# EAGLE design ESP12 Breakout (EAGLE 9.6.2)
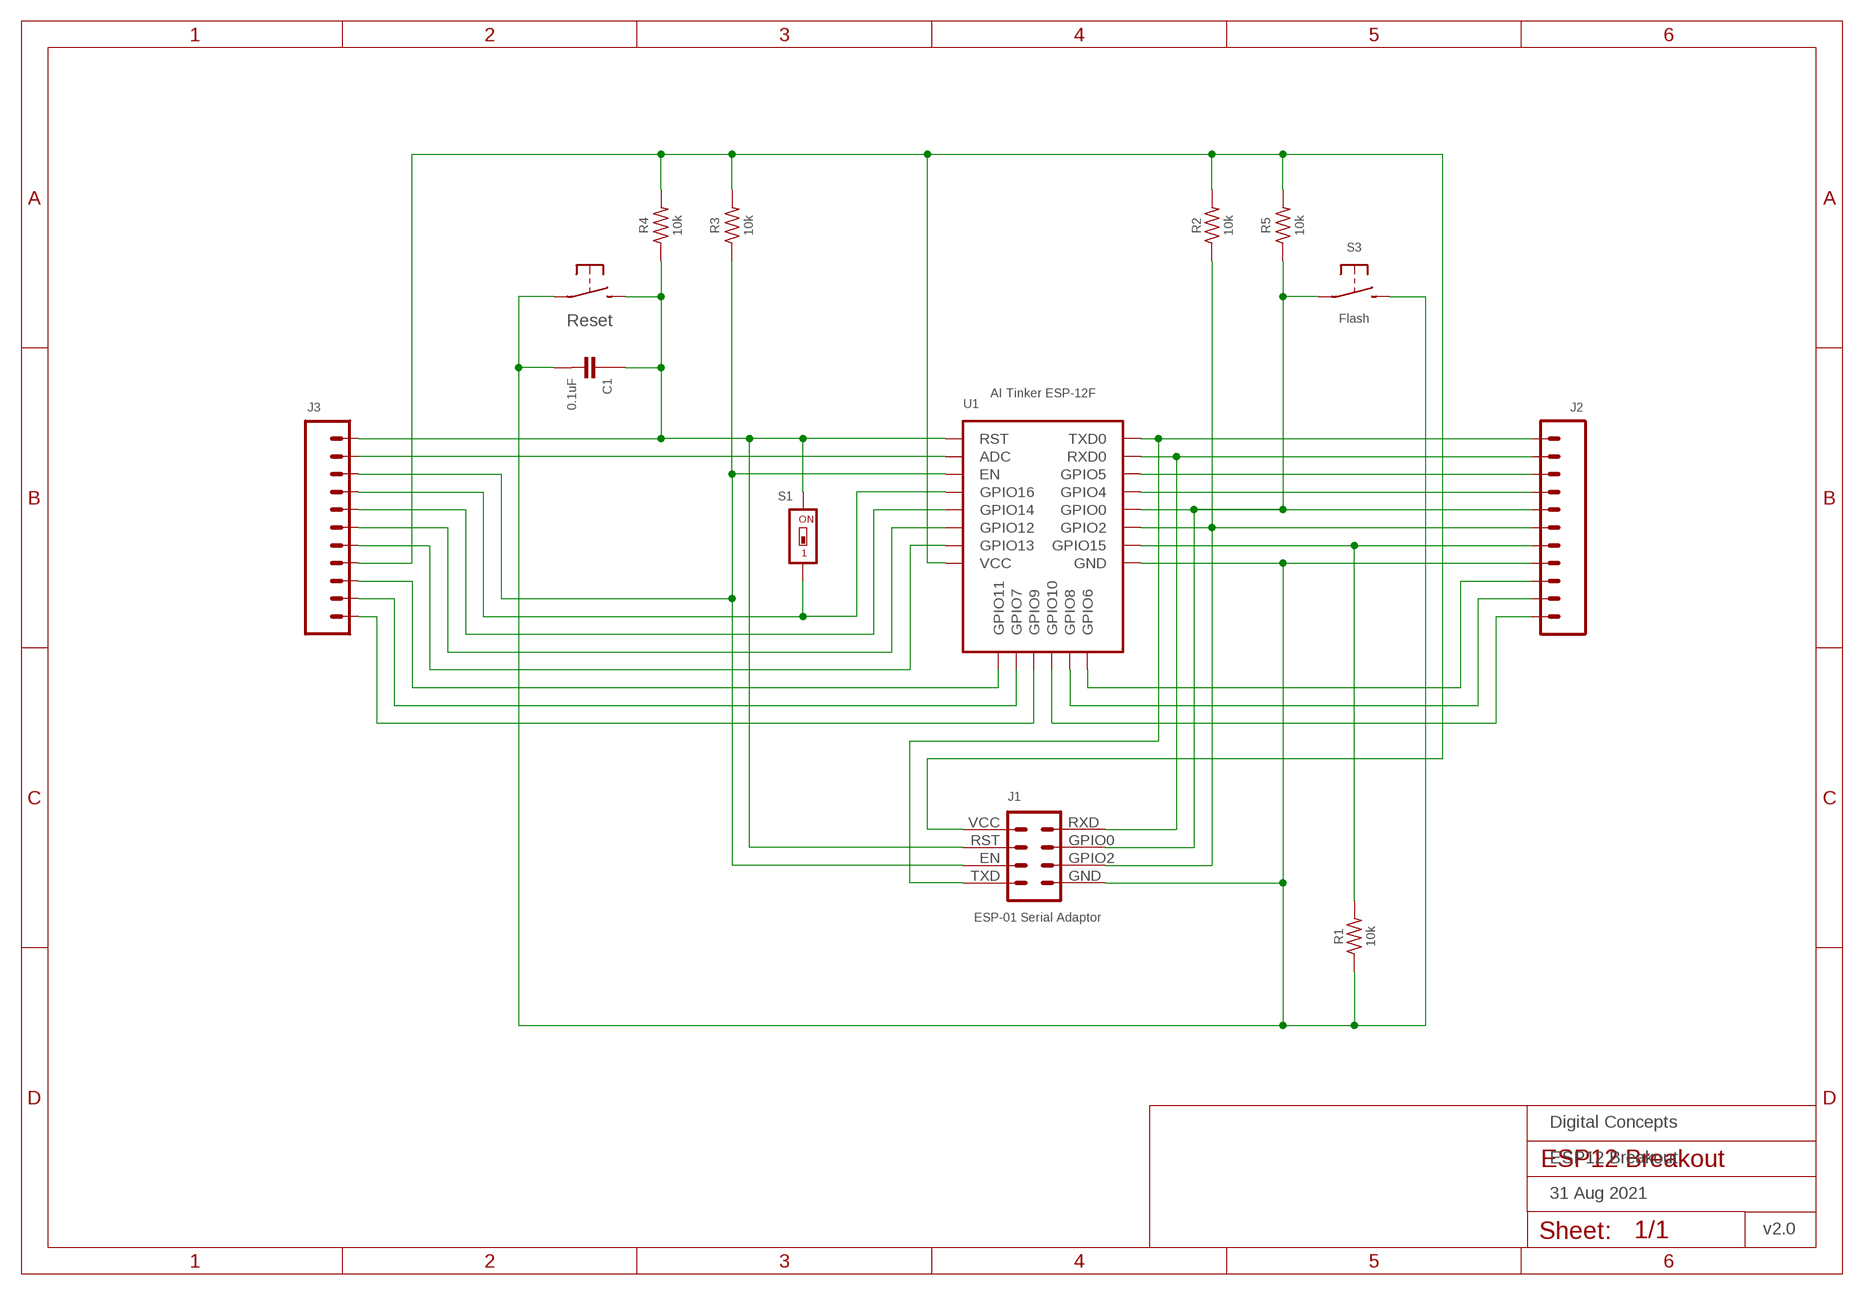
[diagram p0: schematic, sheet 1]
FRAME1 (A4L-LOC): DATE: 31 Aug 2021; OWNER: Digital Concepts; TITLE: ESP12 Breakout; VERSION: v2.0

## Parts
C1  0.1uF  CAPACITOR-0805  [C0805]
J1  ESP-01 Serial Adaptor  ESP-01-SERIAL-ADAPTOR  [CONN_2X4-ESP-01-SERIAL]
J2  HEADER-1X11-GENERIC  [CONN_11-GENERIC]
J3  HEADER-1X11-GENERIC  [CONN_11-GENERIC]
R1  10k  RESISTORR0805  [R0805]
R2  10k  RESISTORR0805  [R0805]
R3  10k  RESISTORR0805  [R0805]
R4  10k  RESISTORR0805  [R0805]
R5  10k  RESISTORR0805  [R0805]
S1  Wake  SWITCH-DIP-SWS001  [SMD-001]
S2  Reset  SWITCH-MOMENTARY-2-PIN  [SWITCH-2-PAD]
S3  Flash  SWITCH-MOMENTARY-2-PIN  [SWITCH-2-PAD]
U1  AI Tinker ESP-12F  ESP-12E/F  [ESP-12E/F]

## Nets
GND: C1.2 J1.GND J2.4 R1.1 S2.P$1(P) S3.P$2(S) U1.GND
N$1: J3.1 U1.GPIO9
N$2: J2.5 R1.2 U1.GPIO15
N$3: J3.7 U1.GPIO14
N$4: C1.1 J1.RST J3.11 R4.1 S1.2 S2.P$2(S) U1.RST
N$5: J3.6 U1.GPIO12
N$6: J3.5 U1.GPIO13
N$7: J3.10 U1.ADC
N$8: J1.EN J3.9 R3.1 U1.EN
N$9: J2.9 U1.GPIO5
N$10: J1.TXD J2.11 U1.TXD0
N$11: J1.GPIO2 J2.6 R2.1 U1.GPIO2
N$12: J2.8 U1.GPIO4
N$13: J1.GPIO0 J2.7 R5.1 S3.P$1(P) U1.GPIO0
N$15: J2.1 U1.GPIO10
N$16: J1.RXD J2.10 U1.RXD0
N$17: J2.3 U1.SCLK(GPIO6)
N$18: J3.8 S1.1 U1.GPIO16
N$19: J2.2 U1.MOSI(GPIO8)
N$22: J3.3 U1.CS0(GPIO11)
N$23: J3.2 U1.MISO(GPIO7)
VCC: J1.VCC J3.4 R2.2 R3.2 R4.2 R5.2 U1.VCC

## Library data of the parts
C1 = digitalconcepts:CAPACITOR-0805: 0805 Capacitor
J1 = digitalconcepts:ESP-01-SERIAL-ADAPTOR: ESP-01 Serial Adpator
J2 J3 = digitalconcepts:HEADER-1X11-GENERIC: Single Row 11-Pin Header
R1-R5 = digitalconcepts:RESISTOR: Resistor; SPICEPREFIX: R
S1 = digitalconcepts:SWITCH-DIP-SWS001: SMD Dip Switch 1 pol.
S2 S3 = digitalconcepts:SWITCH-MOMENTARY-2-PIN: 2 Pin Momentary Switch
U1 = digitalconcepts:ESP-12E/F: AI Thinker ESP-12E/F MCU

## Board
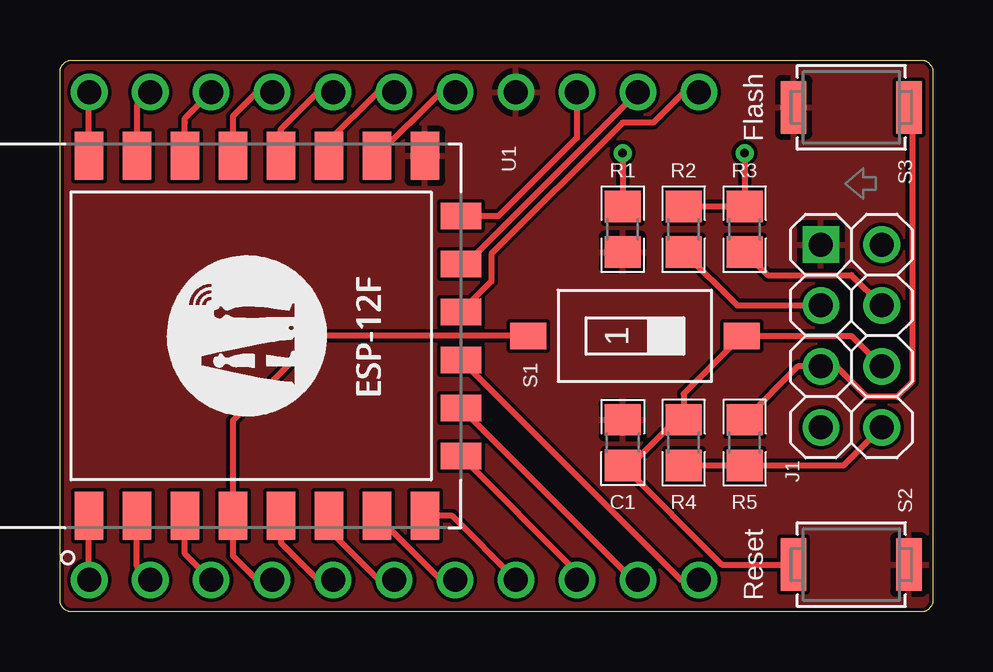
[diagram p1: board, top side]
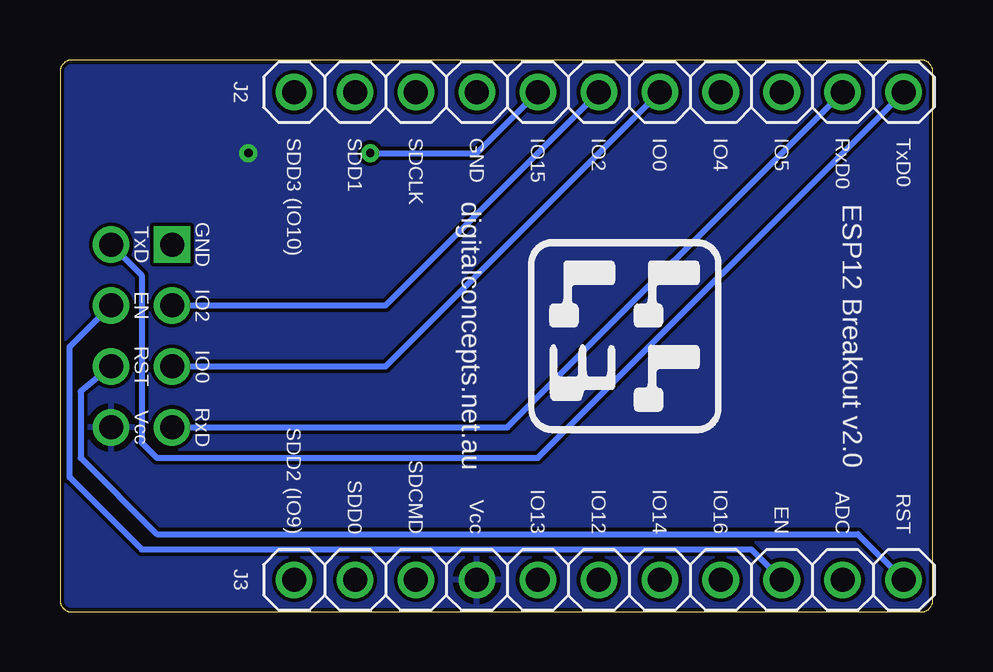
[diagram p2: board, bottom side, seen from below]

Size 36.37 x 23 mm. Coordinates in mm from the lower left corner, seen from the top.
Outline: 88 segments
Copper layers (1*16): Top 0.035mm / dielectric 1.5mm / Bottom 0.035mm
Design rules "default *": minimum track width 6mil, minimum drill 0.35mm, track to track 6mil, track to pad 6mil, pad to pad 6mil, via to via 6mil, smd to smd 6mil, copper to edge 6mil, drill to drill 6mil, minimum pad ring 10mil, minimum via ring 8mil, stop-mask expansion 4mil, vias tented up to drill 0mil, thermal gap 10mil

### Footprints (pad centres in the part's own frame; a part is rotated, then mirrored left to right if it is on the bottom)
C0805 = smd 1.3 x 1.5: 1 -0.95,0; 2 0.95,0
CONN_2X4-ESP-01-SERIAL = drill 1 pad 1.524: EN 2.54,2.54; GPIO0 5.08,0; GPIO2 2.54,0; RST 5.08,2.54; RXD 7.62,0; TXD 0,2.54; VCC 7.62,2.54 | drill 1 pad 1.524 square: GND 0,0
CONN_11-GENERIC = drill 1 pad 1.524: 1 0,0; 2 2.54,0; 3 5.08,0; 4 7.62,0; 5 10.16,0; 6 12.7,0; 7 15.24,0; 8 17.78,0; 9 20.32,0; 10 22.86,0; 11 25.4,0
R0805 = smd 1.3 x 1.5: 1 -0.95,0; 2 0.95,0
SMD-001 = smd 1.1 x 1.5: 1 0,-4.45; 2 0,4.45
SWITCH-2-PAD = smd 1.067 x 2.184: P$1 -2.4,0; P$2 2.4,0
ESP-12E/F = smd 2 x 1.2: ADC -7.5,5; EN -7.5,3; GND 7.5,-7; GPIO0 7.5,-1; GPIO2 7.5,-3; GPIO4 7.5,1; GPIO5 7.5,3; GPIO12 -7.5,-3; GPIO13 -7.5,-5; GPIO14 -7.5,-1; GPIO15 7.5,-5; GPIO16 -7.5,1; RST -7.5,7; RXD0 7.5,5; TXD0 7.5,7; VCC -7.5,-7 | smd 1.1 x 1.7: CS0 -5,-8.5; GPIO9 -1,-8.5; GPIO10 1,-8.5; MISO -3,-8.5; MOSI 3,-8.5; SCLK 5,-8.5

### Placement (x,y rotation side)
C1  23.44,7.06 90 top
J1  31.7,15.31 270 top
J2  26.62,21.66 0 bottom
J3  26.62,1.34 0 bottom
R1  23.44,15.95 90 top
R2  25.98,15.95 90 top
R3  28.52,15.95 90 top
R4  25.98,7.06 270 top
R5  28.52,7.06 270 top
S1  23.95,11.5 270 top
S2  32.97,1.98 180 top
S3  32.97,21.03 180 top
U1  8.2,11.5 90 top

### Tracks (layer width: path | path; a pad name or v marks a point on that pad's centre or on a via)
GND
  pour Top (rank 3): -1.32,24.2 37.41,24.2 37.41,-1.2 -1.32,-1.2
N$1
  Top 0.254: U1.GPIO9 25.86,1.34 J3.1
N$2  (via drill 0.35)
  Top 0.254: U1.GPIO15 15.86,21.66 J2.5 | v23.44,19.12 R1.2
  Bottom 0.254: J2.5 19,19.12 v23.44,19.12
N$3
  Top 0.254: U1.GPIO14 9.2,2.88 10.74,1.34 J3.7
N$4
  Top 0.254: J1.RST 32.97,11.5 S1.2 25.98,9.08 R4.1 25.68,8.01 23.78,6.11 C1.1 27.57,1.98 S2.P$2 | J3.11 1.2,1.36 U1.RST
  Bottom 0.254: J1.RST 35.51,9.19 35.51,6.42 32.33,3.25 3.12,3.25 J3.11
N$5
  Top 0.254: U1.GPIO12 11.2,3.42 13.28,1.34 J3.6
N$6
  Top 0.254: U1.GPIO13 15.86,1.34 J3.5
N$7
  Top 0.254: U1.ADC 3.2,1.9 J3.10
N$8
  Top 0.254: R3.1 29.48,14.04 32.97,14.04 J1.EN | U1.EN 5.2,2.44 J3.9
  Bottom 0.254: J1.EN 35.97,11.04 35.97,5.61 32.97,2.61 7.57,2.61 J3.9
N$9
  Top 0.254: U1.GPIO5 5.2,20.39 5.2,20.57 J2.9
N$10
  Top 0.254: U1.TXD0 1.2,21.65 J2.11
  Bottom 0.254: J1.TXD 32.97,14.04 32.97,7.06 32.33,6.42 16.46,6.42 J2.11
N$11
  Top 0.254: U1.GPIO2 11.2,19.64 13.23,21.66 J2.6 | R2.1 28.21,12.77 J1.GPIO2
  Bottom 0.254: J1.GPIO2 22.81,12.77 J2.6
N$12
  Top 0.254: U1.GPIO4 7.2,20.66 8.2,21.66 J2.8
N$13
  Top 0.254: U1.GPIO0 9.2,20.12 | 9.2,20.12 | 9.2,20.12 10.74,21.66 J2.7 | R5.1 30.75,10.23 J1.GPIO0 32.33,10.23 33.6,8.96 34.87,8.96 35.51,9.6 35.51,20.89 S3.P$1
  Bottom 0.254: J1.GPIO0 22.81,10.23 J2.7
N$15
  Top 0.254: U1.GPIO10 17.97,13.77 17.97,14.92 23.44,20.39 24.71,20.39 25.98,21.66 J2.1
N$16
  Top 0.254: U1.RXD0 3.2,21.11 J2.10
  Bottom 0.254: J1.RXD 17.73,7.69 J2.10
N$17
  Top 0.254: U1.SCLK 18.28,16.5 21.54,19.76 J2.3
N$18
  Top 0.254: S1.1 10.74,11.5 7.2,7.96 U1.GPIO16 7.2,2.34 8.2,1.34 J3.8
N$19
  Top 0.254: J2.2 16.92,14.5 U1.MOSI
N$22
  Top 0.254: U1.CS0 21.54,1.67 J3.3
N$23
  Top 0.254: U1.MISO 23.86,1.34 J3.2
VCC  (via drill 0.35)
  Top 0.254: U1.VCC 16.34,4 J3.4 | R4.2 R5.2 32.65,6.11 J1.VCC | R2.2 R3.2 v28.52,19.12
  pour Bottom (rank 3): -0.69,23.57 36.78,23.57 36.78,-0.56 -0.69,-0.56

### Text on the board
bPlace: TxD0 | RxD0 | IO5 | IO4 | IO0 | IO2 | IO15 | GND | SDCLK | SDD1 | SDD3 (IO10) | GND | TxD | IO2 | EN | ESP12 Breakout v2.0 | digitalconcepts.net.au | IO0 | RST | RxD | Vcc | RST | ADC | EN | IO16 | IO14 | IO12 | IO13 | Vcc | SDCMD | SDD0 | SDD2 (IO9)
